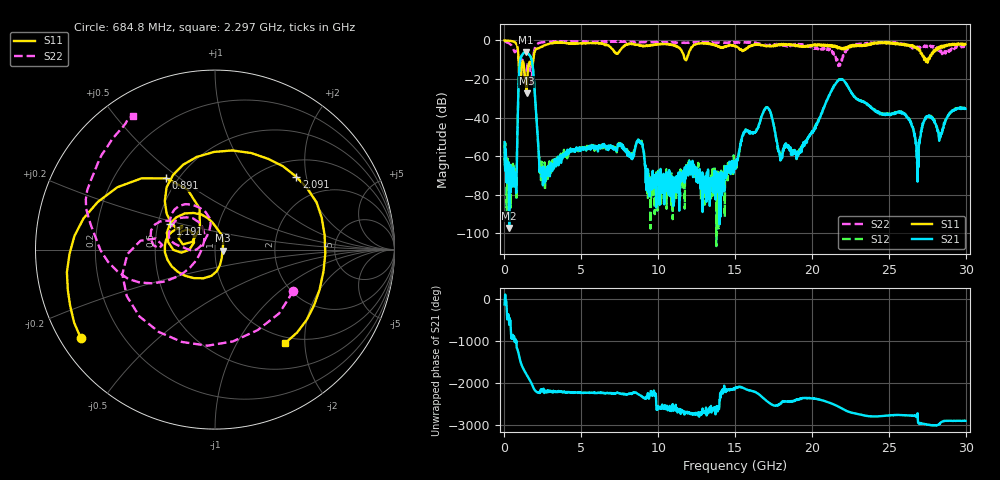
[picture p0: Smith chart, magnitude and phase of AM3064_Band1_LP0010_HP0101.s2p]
# Hz S DB R 50.0
!freq dBS11 angS11 dBS21 angS21 dBS12 angS12 dBS22 angS22
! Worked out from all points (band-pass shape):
!   1600 points, 10 MHz to 29.98 GHz, reference 50 ohm
!   highest |S21| = -5.98 dB at 1.378 GHz (marker M1); lowest = -97.3 dB at 309.9 MHz (marker M2)
!   |S21| within 3 dB of the highest: 1.066 GHz to 1.724 GHz (657.6 MHz wide, 47.1 % of centre)
!   lowest |S11| = -27.5 dB at 1.435 GHz (marker M3), VSWR 1.09, Z = 54.4 - j0.695 ohm
!   |S11| at or under -10 dB: 916.8 MHz to 1.877 GHz (960.5 MHz wide, 68.8 % of centre); 11.75 GHz to 11.84 GHz (89.42 MHz wide, 0.758 % of centre); 27.39285 GHz to 27.46088 GHz (68.02 MHz wide, 0.248 % of centre)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
!   |S22| runs from -22.9 to -0.3 dB; largest |S21 - S12| = 0.0054
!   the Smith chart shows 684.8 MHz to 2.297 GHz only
!   S11 on the Smith chart (normalised r, x): 684.8 MHz: 0.06, -0.30; 891 MHz: 0.43, +0.45; 1.191 GHz: 0.58, +0.18; 2.091 GHz: 1.36, +1.75; 2.297 GHz: 0.90, -1.63
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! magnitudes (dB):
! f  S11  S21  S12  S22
! 10 MHz  0.0  -52.7  -54.2  -0.3
! 309.9 MHz  -0.2  -97.3  -66.5  -1.6
! 684.8 MHz  -1.0  -68.5  -67.3  -6.1
! 891 MHz  -6.4  -30.3  -30.3  -7.6
! 1.191 GHz  -10.8  -7.1  -7.1  -10.4
! 1.378 GHz  -21.2  -6.0  -6.0  -19.9
! 1.435 GHz  -27.5  -6.1  -6.0  -16.2
! 1.791 GHz  -13.1  -10.9  -10.9  -17.5
! 2.091 GHz  -4.3  -41.5  -41.3  -2.1
! 2.297 GHz  -3.7  -67.0  -68.6  -1.2
! 5.015 GHz  -1.4  -56.0  -56.2  -0.7
! 8.782 GHz  -2.7  -52.2  -52.7  -0.9
! 10 GHz  -2.0  -73.1  -73.6  -0.9
! 15 GHz  -2.9  -66.6  -65.4  -1.3
! 17.03 GHz  -3.1  -34.7  -34.9  -2.7
! 17.95 GHz  -2.3  -62.3  -60.9  -1.9
! 19.99 GHz  -2.9  -47.3  -47.6  -3.4
! 21.83 GHz  -3.9  -20.3  -20.3  -13.1
! 25 GHz  -1.0  -38.3  -38.2  -1.2
! 26.87 GHz  -4.4  -73.3  -65.6  -3.2
! 27.49 GHz  -10.0  -39.6  -39.5  -3.0
! 29.98 GHz  -1.8  -35.5  -35.6  -3.3
